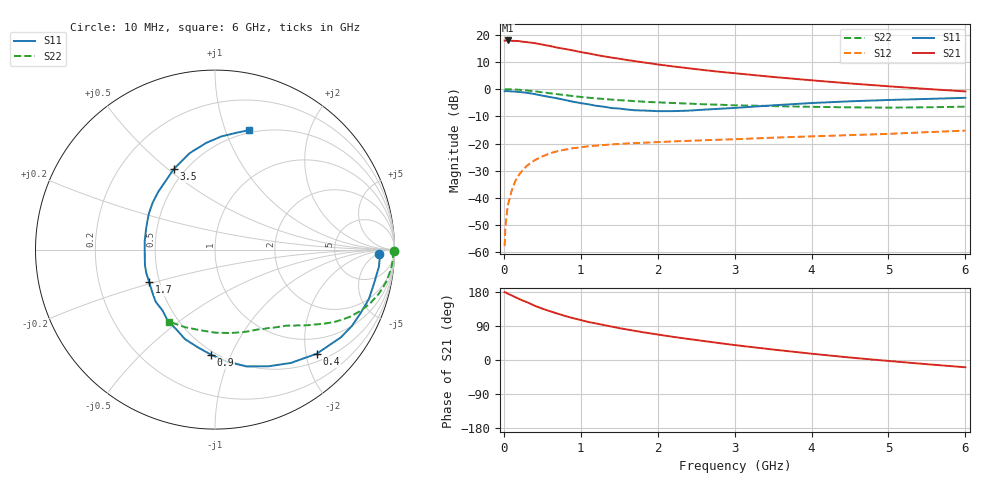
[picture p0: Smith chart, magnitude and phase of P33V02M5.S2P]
! SIEMENS Small Signal Semiconductors
! BFP181
! Si NPN RF Bipolar Junction Transistor in SOT143
! VCE = 3 V  IC = 2.5 mA
! Common Emitter S-Parameters:  March  1996
# GHz  S  MA  R  50
!  f  S11  S21  S12  S22
! GHz  MAG  ANG  MAG  ANG  MAG  ANG  MAG  ANG
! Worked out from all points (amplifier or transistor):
!   36 points, 10 MHz to 6 GHz, reference 50 ohm
!   highest |S21| = 17.9 dB at 50 MHz (marker M1)
!   |S21| within 3 dB of that: start of sweep to 770 MHz
!   unconditionally stable (mu >= 1): 2.258 GHz to end of sweep
!   at 250 MHz: K = 0.14, MSG = 23.5 dB, |S12| = -29.7 dB
!   at 1.4 GHz: K = 0.71, MSG = 16.0 dB, |S12| = -20.3 dB
!   at 6 GHz: K = 1.12, MAG = 5.1 dB, |S12| = -15.3 dB
!   S11 on the Smith chart (normalised r, x): 10 MHz: 21, -6; 400 MHz: 0.65, -2.21; 900 MHz: 0.47, -0.85; 1.7 GHz: 0.44, -0.19; 3.5 GHz: 0.44, +0.52; 6 GHz: 0.47, +1.21
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0.01  0.9161 -1.4  7.784 179.1  0.0013 82.3  0.9966 -0.5
0.02  0.9194 -2.1  7.767 178.6  0.0029 88.9  0.9907 -1.0
0.05  0.9184 -5.9  7.84 175.2  0.0071 89.7  0.9924 -2.7
0.1  0.906 -11.9  7.703 170.5  0.0134 81.7  0.9888 -5.3
0.2  0.8852 -23.5  7.629 161.0  0.0271 75.2  0.9712 -10.5
0.25  0.8731 -29.2  7.408 156.4  0.0328 73.1  0.9585 -12.9
0.3  0.8553 -34.8  7.302 152.6  0.039 70.1  0.9451 -15.1
0.4  0.811 -45.7  7.007 143.3  0.0493 63.9  0.9122 -19.5
0.5  0.7599 -56.2  6.585 135.5  0.058 58.6  0.8754 -23.2
0.6  0.715 -65.4  6.205 128.7  0.066 53.7  0.8406 -26.4
0.7  0.6741 -74.9  5.764 122.2  0.0725 50.1  0.806 -29.1
0.8  0.6294 -83.7  5.461 116.0  0.0773 46.2  0.7751 -31.4
0.9  0.5863 -92.1  5.139 110.4  0.0821 43.2  0.744 -33.5
1.1  0.5263 -108.5  4.535 100.4  0.0892 38.3  0.695 -36.9
1.4  0.4484 -130.6  3.801 88.2  0.0964 33.2  0.6422 -41.3
1.7  0.4089 -153.7  3.271 77.0  0.1016 29.8  0.6008 -44.8
2.2  0.3945 173.3  2.615 61.1  0.1093 26.1  0.5553 -50.9
2.8  0.4351 142.8  2.086 44.6  0.1176 23.2  0.5167 -59.0
3.5  0.5037 117.2  1.674 27.6  0.1281 20.8  0.4881 -70.0
4.5  0.5971 94.6  1.272 6.5  0.1427 16.8  0.4627 -89.9
5.5  0.6603 79.9  1.007 -11.1  0.1617 13.9  0.4638 -111.4
6  0.6916 74.2  0.908 -19.2  0.1727 11.4  0.4755 -122.5
